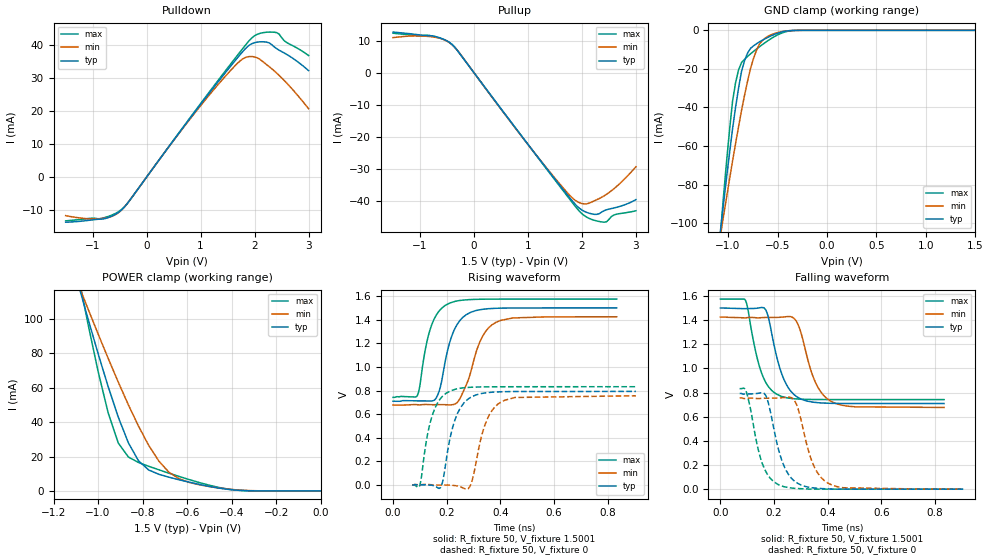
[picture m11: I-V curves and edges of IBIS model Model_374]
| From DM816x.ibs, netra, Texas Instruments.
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| Model based on original model for BSHTLTCSCDDVGPBFZ
|   Sub model FASTEST_9MA_5PER_N_1P5
[model]   Model_374
|[Description]  1.5V-3-STATE-X-FASTEST, 9MA, +-5%
|[Input Load]
|[Output Drive] FASTEST, 9MA
|Voltage   1.5V
|Mode   3-STATE
Model_type   3-state
Polarity   Non-Inverting
Enable   Active-Low
Cref =  15.0000pF
Rref =  100.0000M
Vref =  0V
Vmeas =  0.75005
C_comp   1.5249p   1.4275p   1.6205p
[Model Spec]
[Temperature Range]   25   125   -40
[Voltage Range]   1.5   1.425   1.575
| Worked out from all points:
|   slope of the pulldown table from 0 to 0.225 V, typ, clamps not added: 44.4 ohm
|   slope of the pullup table from 0 to 0.225 V, typ, clamps not added: 44.4 ohm
|   GND clamp passes 1 mA (typ) near -0.47 V on its own axis
|   POWER clamp passes 1 mA (typ) near -0.42 V on its own axis
|   rising waveform, R_fixture 50, V_fixture 1.5001: 20-80 % time 54.4ps typ, 69.3ps min, 49.6ps max; typ from 0.71 V to 1.5 V
|   rising waveform, R_fixture 50, V_fixture 0: 20-80 % time 51.8ps typ, 55.5ps min, 48.1ps max; typ from 0 V to 0.793 V
|   falling waveform, R_fixture 50, V_fixture 1.5001: 20-80 % time 59ps typ, 65.2ps min, 54.9ps max; typ from 1.5 V to 0.709 V
|   falling waveform, R_fixture 50, V_fixture 0: 20-80 % time 57.2ps typ, 60.8ps min, 52.6ps max; typ from 0.793 V to 0 V
[POWER_clamp]
-1.5V     321.7mA    260.6mA    415.9mA
-1.076V   114.2mA    115.8mA    116.9mA
-1.061V   107.2mA    110.9mA    107.1mA
-954.6mV  60.59mA    77.06mA    45.35mA
-909.2mV  42.85mA    63.21mA    27.81mA
-863.7mV  27.9mA     49.99mA    19.69mA
-818.2mV  17.49mA    37.63mA    16.52mA
-772.8mV  12.19mA    26.53mA    14.33mA
-681.9mV  7.985mA    10.89mA    10.33mA
-590.9mV  5.094mA    4.955mA    6.6mA
-363.7mV  298.5uA    465.2uA    297.6uA
0V        1.518nA    24.08nA    367.8pA
[Pulldown]
-1.5V     -13.72mA   -11.73mA   -13.31mA
-863.7mV  -12.8mA    -12.65mA   -12.66mA
-500mV    -10.46mA   -10.55mA   -10.29mA
-318.2mV  -7.172mA   -7.186mA   -7.182mA
1.046V    23.05mA    22.61mA    23.31mA
1.591V    34.39mA    33mA       35.06mA
1.818V    38.82mA    36.24mA    39.81mA
1.955V    40.55mA    36.61mA    42.37mA
2.091V    41.08mA    35.83mA    43.61mA
2.273V    40.74mA    33.5mA     44.04mA
2.364V    39.55mA    32.26mA    43.99mA
3V        32.34mA    20.77mA    36.92mA
[Pullup]
-1.5V     12.66mA    10.94mA    12.31mA
-818.2mV  11.55mA    11.26mA    11.58mA
-590.9mV  10.61mA    10.52mA    10.54mA
-409.1mV  8.836mA    8.777mA    8.84mA
1.227V    -27.25mA   -27.19mA   -27.38mA
1.727V    -37.96mA   -37.32mA   -38.38mA
1.909V    -41.55mA   -40.1mA    -42.29mA
2.046V    -43.18mA   -40.84mA   -44.51mA
2.227V    -44.08mA   -39.9mA    -45.94mA
2.409V    -42.96mA   -38.35mA   -46.53mA
2.591V    -42.11mA   -36.14mA   -44.31mA
3V        -39.5mA    -29.28mA   -42.98mA
[GND_clamp]
-1.5V     -310.1mA   -250.5mA   -402.5mA
-1.076V   -103.6mA   -106.2mA   -105.2mA
-1.046V   -89.81mA   -96.36mA   -86.02mA
-954.6mV  -51.22mA   -67.87mA   -36.88mA
-924.3mV  -40.08mA   -58.86mA   -27.29mA
-863.7mV  -21.24mA   -41.56mA   -16.73mA
-833.4mV  -15.8mA    -33.75mA   -15.03mA
-772.8mV  -9.345mA   -19.75mA   -12.19mA
-712.2mV  -6.928mA   -10.35mA   -9.704mA
-621.3mV  -4.261mA   -3.896mA   -6.225mA
-409.1mV  -337.1uA   -289.1uA   -618.9uA
1.5V      1.518nA    257.2nA    299pA
[Ramp]
dV/dt_f   0.636912/93.554374p   0.602712/0.10536803n   0.668424/85.90732p
dV/dt_r   0.656732/84.321741p  0.6328336/91.397271p  0.6817744/76.969402p
R_load = 50
[Rising Waveform]
R_fixture = 50
V_fixture = 1.5001
V_fixture_min = 1.425
V_fixture_max = 1.575
0s        709.9mV    677.4mV    742.6mV
91.6ps    712.8mV    680.1mV    763.7mV
126.7ps   712.1mV    682.2mV    1.218V
156.9ps   725.4mV    680.3mV    1.422V
176.1ps   828.5mV    680.9mV    1.485V
211.6ps   1.211V     679.2mV    1.542V
273.6ps   1.444V     852.8mV    1.569V
323.4ps   1.484V     1.212V     1.573V
382.2ps   1.497V     1.376V     1.575V
833.3ps   1.5V       1.425V     1.575V
[Rising Waveform]
R_fixture = 50
V_fixture = 0
V_fixture_min = 0
V_fixture_max = 0
71.67ps   0V         0V         0V
98.42ps   2.274mV    2.513mV    -10.41mV
133.7ps   0V         4.106mV    484.1mV
176.9ps   -21.33mV   0V         732.6mV
213.2ps   404.1mV    0V         796.7mV
239.5ps   603.5mV    -7.751mV   815.3mV
282.7ps   733.3mV    -24.98mV   827mV
343.2ps   780mV      513.8mV    831.4mV
415.5ps   790.8mV    717.7mV    832.4mV
905ps     793mV      756.2mV    832.8mV
[Falling Waveform]
R_fixture = 50
V_fixture = 1.5001
V_fixture_min = 1.425
V_fixture_max = 1.575
0s        1.501V     1.425V     1.575V
92.81ps   1.495V     1.419V     1.566V
135.8ps   1.499V     1.42V      1.098V
163.1ps   1.501V     1.422V     911.2mV
179.5ps   1.417V     1.422V     847.6mV
226.5ps   968.3mV    1.425V     769.2mV
282.3ps   770mV      1.393V     747.9mV
354.6ps   718.5mV    882mV      742.9mV
410.4ps   711.2mV    729.9mV    742.2mV
833.3ps   709.3mV    676.9mV    741.9mV
[Falling Waveform]
R_fixture = 50
V_fixture = 0
V_fixture_min = 0
V_fixture_max = 0
71.67ps   793mV      756.9mV    832.6mV
96.48ps   788.4mV    751.1mV    807.5mV
143.5ps   795.1mV    750.7mV    305.5mV
168.4ps   778.4mV    753.4mV    150.1mV
216.6ps   329.1mV    755.4mV    36.55mV
245.1ps   154.5mV    761mV      16.88mV
276.8ps   65.73mV    732.5mV    6.994mV
342.4ps   11.44mV    223.5mV    0V
401.4ps   2.673mV    49.23mV    0V
905ps     0V         0V         0V
